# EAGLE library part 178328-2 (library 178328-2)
TE Connectivity D-3000 Series, 3.81mm Pitch 20 Way Straight PCB Header, Solder Termination Source: Datasheet
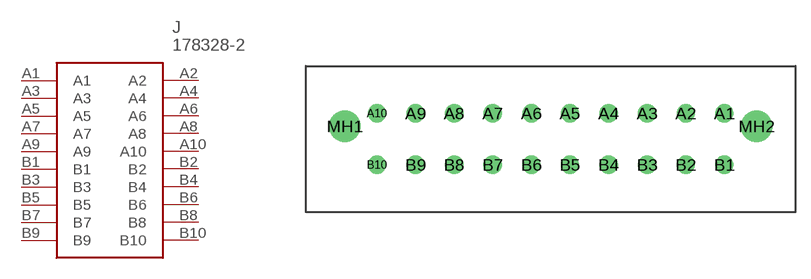
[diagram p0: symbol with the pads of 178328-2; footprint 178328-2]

Designator prefix J

## 178328-2 (Description: TE Connectivity D-3000 Series, 3.81mm Pitch 20 Way Straight PCB Header, Solder Termination; Height: mm; Manufacturer_Name: TE Connectivity; Manufacturer_Part_Number: 178328-2; Mouser_Part_Number: 571-178328-2; Mouser_Price-Stock: https://www.mouser.com/Search/Refine.aspx?Keyword=571-178328-2; RS_Part_Number: 6803460; RS_Price-Stock: http://uk.rs-online.com/web/p/products/6803460)  [178328-2]
A1  A1
A2  A2
A3  A3
A4  A4
A5  A5
A6  A6
A7  A7
A8  A8
A9  A9
A10  A10
B1  B1
B2  B2
B3  B3
B4  B4
B5  B5
B6  B6
B7  B7
B8  B8
B9  B9
B10  B10

## Footprint 178328-2 (pad centres in mm)
178328-2
drill 1.2 pad 1.8: A1 17.145,2.54; A2 13.335,2.54; A3 9.525,2.54; A4 5.715,2.54; A5 1.905,2.54; A6 -1.905,2.54; A7 -5.715,2.54; A8 -9.525,2.54; A9 -13.335,2.54; A10 -17.145,2.54; B1 17.145,-2.54; B2 13.335,-2.54; B3 9.525,-2.54; B4 5.715,-2.54; B5 1.905,-2.54; B6 -1.905,-2.54; B7 -5.715,-2.54; B8 -9.525,-2.54; B9 -13.335,-2.54; B10 -17.145,-2.54
drill 2.1 pad 3: MH1 -20.32,1.27; MH2 20.32,1.27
